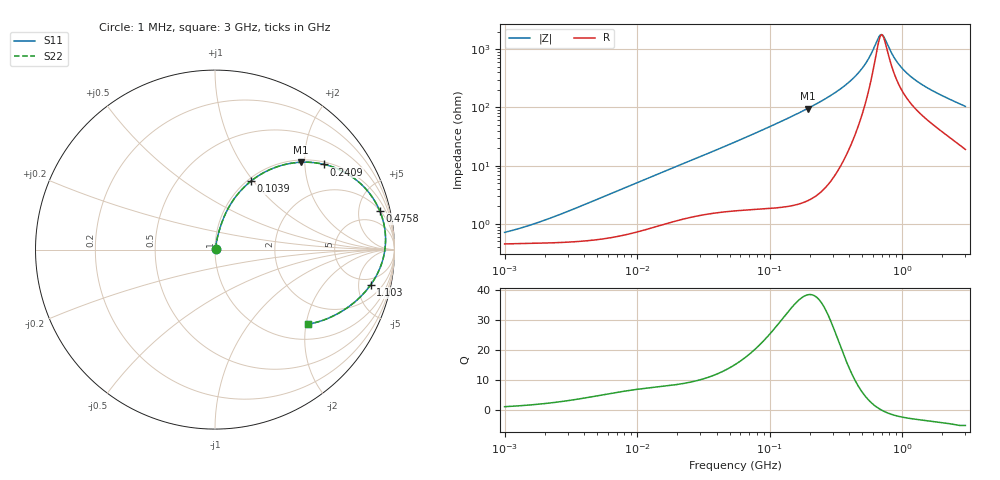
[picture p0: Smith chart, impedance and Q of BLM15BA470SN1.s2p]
! BLM15BA470SN1
# Hz S RI R 50
!Freq.(Hz) S11(Real) S11(Imag) S21(Real) S21(Imag) S12(Real) S12(Imag) S22(Real) S22(Imag)
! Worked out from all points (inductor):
!   401 points, 1 MHz to 3 GHz, reference 50 ohm
!   read as one part in series: L = 83.2 nH near 2.775 MHz
!   highest Q = 38.3 at 193.3 MHz (marker M1), where L = 78.8 nH
!   self-resonance near 705.5 MHz
!   S11 on the Smith chart (normalised r, x): 1 MHz: 1.01, +0.01; 103.9 MHz: 1.04, +0.97; 240.9 MHz: 1.07, +2.51; 475.8 MHz: 2.09, +8.14; 1.103 GHz: 3.73, -7.00; 3 GHz: 1.38, -2.05
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1000000  0.00455 0.0055  0.9954 -0.0055  0.9954 -0.0055  0.00455 0.0055
1786863  0.00473 0.00942  0.9953 -0.00942  0.9953 -0.00942  0.00473 0.00942
3823119  0.00542 0.0197  0.9946 -0.0197  0.9946 -0.0197  0.00542 0.0197
1.461624e7  0.0143 0.0712  0.9857 -0.0712  0.9857 -0.0712  0.0143 0.0712
3.00453e7  0.0331 0.1363  0.9669 -0.1363  0.9669 -0.1363  0.0331 0.1363
5.477226e7  0.0745 0.2318  0.9255 -0.2318  0.9255 -0.2318  0.0745 0.2318
1.039275e8  0.2001 0.3814  0.7999 -0.3814  0.7999 -0.3814  0.2001 0.3814
1.403209e8  0.3138 0.4492  0.6862 -0.4492  0.6862 -0.4492  0.3138 0.4492
1.93289e8  0.4789 0.4867  0.5211 -0.4867  0.5211 -0.4867  0.4789 0.4867
2.094008e8  0.5254 0.4865  0.4746 -0.4865  0.4746 -0.4865  0.5254 0.4865
2.408952e8  0.6085 0.4745  0.3915 -0.4745  0.3915 -0.4745  0.6085 0.4745
3.523638e8  0.8149 0.364  0.1851 -0.364  0.1851 -0.364  0.8149 0.364
4.75755e8  0.9185 0.2147  0.0815 -0.2147  0.0815 -0.2147  0.9185 0.2147
5.583748e8  0.9442 0.126  0.0558 -0.126  0.0558 -0.126  0.9442 0.126
6.553423e8  0.95 0.0385  0.05 -0.0385  0.05 -0.0385  0.95 0.0385
6.821091e8  0.9486 0.0174  0.0514 -0.0174  0.0514 -0.0174  0.9486 0.0174
7.243229e8  0.9446 -0.0136  0.0554 0.0136  0.0554 0.0136  0.9446 -0.0136
8.005644e8  0.9332 -0.0627  0.0668 0.0627  0.0668 0.0627  0.9332 -0.0627
9.209708e8  0.9091 -0.1256  0.0909 0.1256  0.0909 0.1256  0.9091 -0.1256
1.10276e9  0.8675 -0.1962  0.1325 0.1962  0.1325 0.1962  0.8675 -0.1962
1.645649e9  0.7482 -0.3159  0.2518 0.3159  0.2518 0.3159  0.7482 -0.3159
3e9  0.5181 -0.4154  0.4819 0.4154  0.4819 0.4154  0.5181 -0.4154
